FUNCTION "DIALOGO CON AP&T" : VOID
TITLE =Comunicazione AP&T
AUTHOR : D_T
FAMILY : DESTACK
NAME : COMUN
VERSION : 0.1


VAR_TEMP
  Klaschka_Alto : BOOL ;	//Klaschka Alto x Sicurezza movimentazione SMC
  BraccioAPT_FI : BOOL ;	//Braccio AP&T Fuori Ingombro da Pressa
END_VAR
BEGIN
NETWORK
TITLE =Per AP&T: Accensione motori
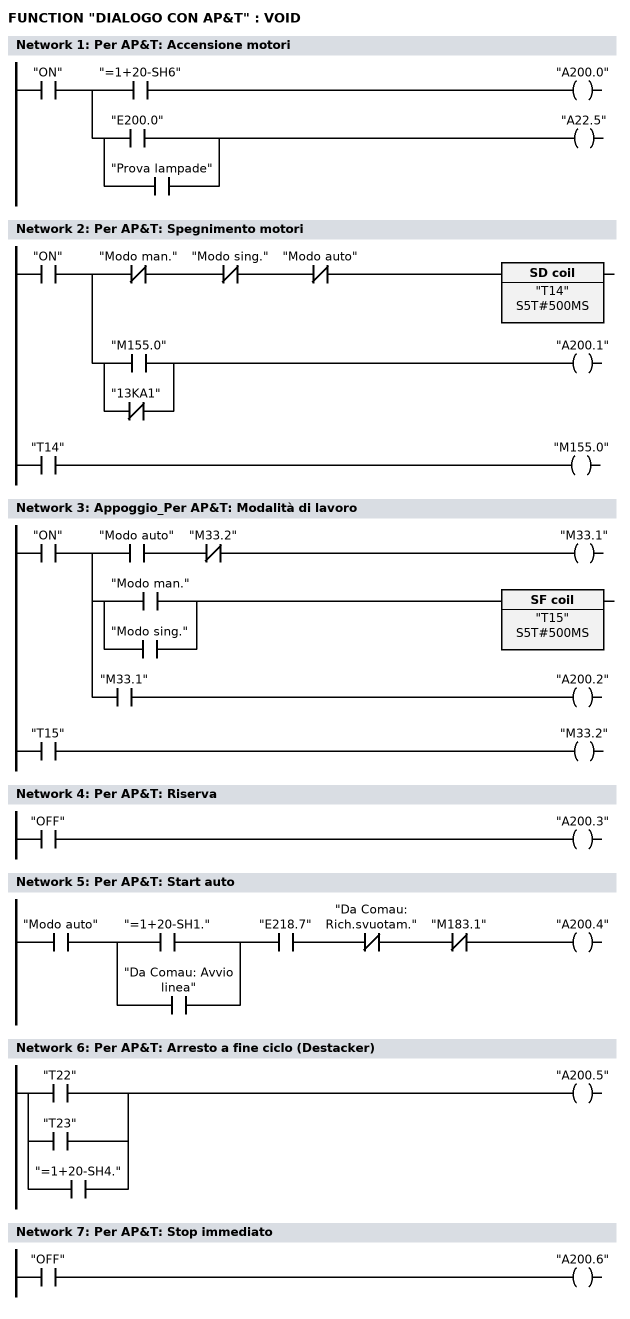
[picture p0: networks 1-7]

      U     "ON";
      =     L      1.0;
      U     L      1.0;
      U     "=1+20-SH6";
      =     "A200.0";
      U     L      1.0;
      U(    ;
      O     "E200.0";
      O     "Prova lampade";
      )     ;
      =     "A22.5";
NETWORK
TITLE =Per AP&T: Spegnimento motori

      U     "ON";
      =     L      1.0;
      U     L      1.0;
      UN    "Modo man.";
      UN    "Modo sing.";
      UN    "Modo auto";
      L     S5T#500MS;
      SE    "T14";
      NOP   0;
      NOP   0;
      NOP   0;
      U     "T14";
      =     "M155.0";
      U     L      1.0;
      U(    ;
      O     "M155.0";
      ON    "13KA1";
      )     ;
      =     "A200.1";
NETWORK
TITLE =Appoggio_Per AP&T: Modalità di lavoro

      U     "ON";
      =     L      1.0;
      U     L      1.0;
      U     "Modo auto";
      UN    "M33.2";
      =     "M33.1";
      U     L      1.0;
      U(    ;
      O     "Modo man.";
      O     "Modo sing.";
      )     ;
      L     S5T#500MS;
      SA    "T15";
      NOP   0;
      NOP   0;
      NOP   0;
      U     "T15";
      =     "M33.2";
      U     L      1.0;
      U     "M33.1";
      =     "A200.2";
NETWORK
TITLE =Per AP&T: Riserva

      U     "OFF";
      =     "A200.3";
NETWORK
TITLE =Per AP&T: Start auto

      U     "Modo auto";
      U(    ;
      O     "=1+20-SH1.";
      O     "Da Comau: Avvio linea";
      )     ;
      U     "E218.7";
      UN    "Da Comau: Rich.svuotam.";
      UN    "M183.1";
      =     "A200.4";
NETWORK
TITLE =Per AP&T: Arresto a fine ciclo (Destacker)

      O     "T22";
      O     "T23";
      O     "=1+20-SH4.";
      =     "A200.5";
NETWORK
TITLE =Per AP&T: Stop immediato

      U     "OFF";
      =     "A200.6";
NETWORK
TITLE =Per AP&T: Vai in posizione di cambio tooling

      U     "ON";
      =     L      1.0;
      U     L      1.0;
      U(    ;
      U     "AP&T in Manuale";
      U     "M130.5";
      O     ;
      U     "AP&T in Automatico";
      U     "Cambio produz. in corso";
      U     "Cambio prod.: Passo 7";
      )     ;
      =     L      1.1;
      U(    ;
      U     L      1.1;
      U     "Gruppi a riposo";
      U     "Magneti Indietro";
      UN    "Retrofitt. Ripari x AP&T";
      UN    "E200.1";
      L     S5T#2S;
      SE    "T59";
      NOP   0;
      NOP   0;
      NOP   0;
      U     "T59";
      )     ;
      FP    "M269.0";
      S     "A200.7";
      U     L      1.1;
      BLD   102;
      =     "Contr.gruppi a riposo";
      U     L      1.0;
      U     "A200.7";
      L     S5T#4S;
      SE    "T45";
      NOP   0;
      NOP   0;
      NOP   0;
      U     "T45";
      R     "A200.7";
NETWORK
TITLE =Per AP&T: Reset allarmi
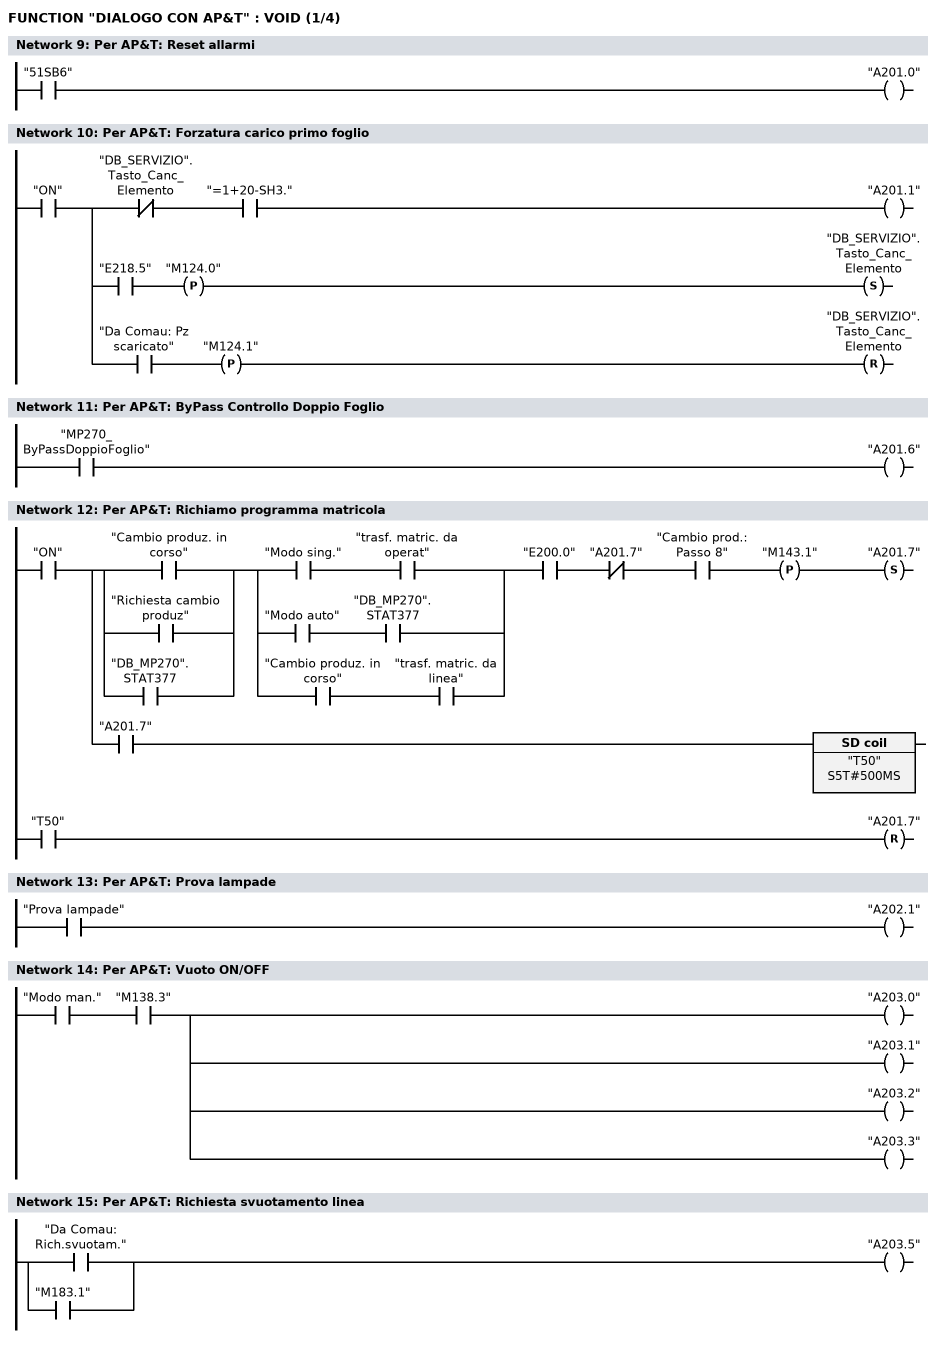
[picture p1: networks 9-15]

      U     "51SB6";
      =     "A201.0";
NETWORK
TITLE =Per AP&T: Forzatura carico primo foglio

      U     "ON";
      =     L      1.0;
      U     L      1.0;
      UN    "DB_SERVIZIO".Tasto_Canc_Elemento;
      U     "=1+20-SH3.";
      =     "A201.1";
      U     L      1.0;
      U     "E218.5";
      FP    "M124.0";
      S     "DB_SERVIZIO".Tasto_Canc_Elemento;
      U     L      1.0;
      U     "Da Comau: Pz scaricato";
      FP    "M124.1";
      R     "DB_SERVIZIO".Tasto_Canc_Elemento;
NETWORK
TITLE =Per AP&T: ByPass Controllo Doppio Foglio

      U     "MP270_ByPassDoppioFoglio";
      =     "A201.6";
NETWORK
TITLE =Per AP&T: Richiamo programma matricola

      U     "ON";
      =     L      1.0;
      U     L      1.0;
      U(    ;
      O     "Cambio produz. in corso";
      O     "Richiesta cambio produz";
      O     "DB_MP270".STAT377;
      )     ;
      U(    ;
      U     "Modo sing.";
      U     "trasf. matric. da operat";
      O     ;
      U     "Modo auto";
      U     "DB_MP270".STAT377;
      O     ;
      U     "Cambio produz. in corso";
      U     "trasf. matric. da linea";
      )     ;
      U     "E200.0";
      UN    "A201.7";
      U     "Cambio prod.: Passo 8";
      FP    "M143.1";
      S     "A201.7";
      U     L      1.0;
      U     "A201.7";
      L     S5T#500MS;
      SE    "T50";
      NOP   0;
      NOP   0;
      NOP   0;
      U     "T50";
      R     "A201.7";
NETWORK
TITLE =Per AP&T: Prova lampade

      U     "Prova lampade";
      =     "A202.1";
NETWORK
TITLE =Per AP&T: Vuoto ON/OFF

      U     "Modo man.";
      U     "M138.3";
      =     "A203.0";
      =     "A203.1";
      =     "A203.2";
      =     "A203.3";
NETWORK
TITLE =Per AP&T: Richiesta svuotamento linea

      O     "Da Comau: Rich.svuotam.";
      O     "M183.1";
      =     "A203.5";
NETWORK
TITLE =Per AP&T: Richiesta apertura
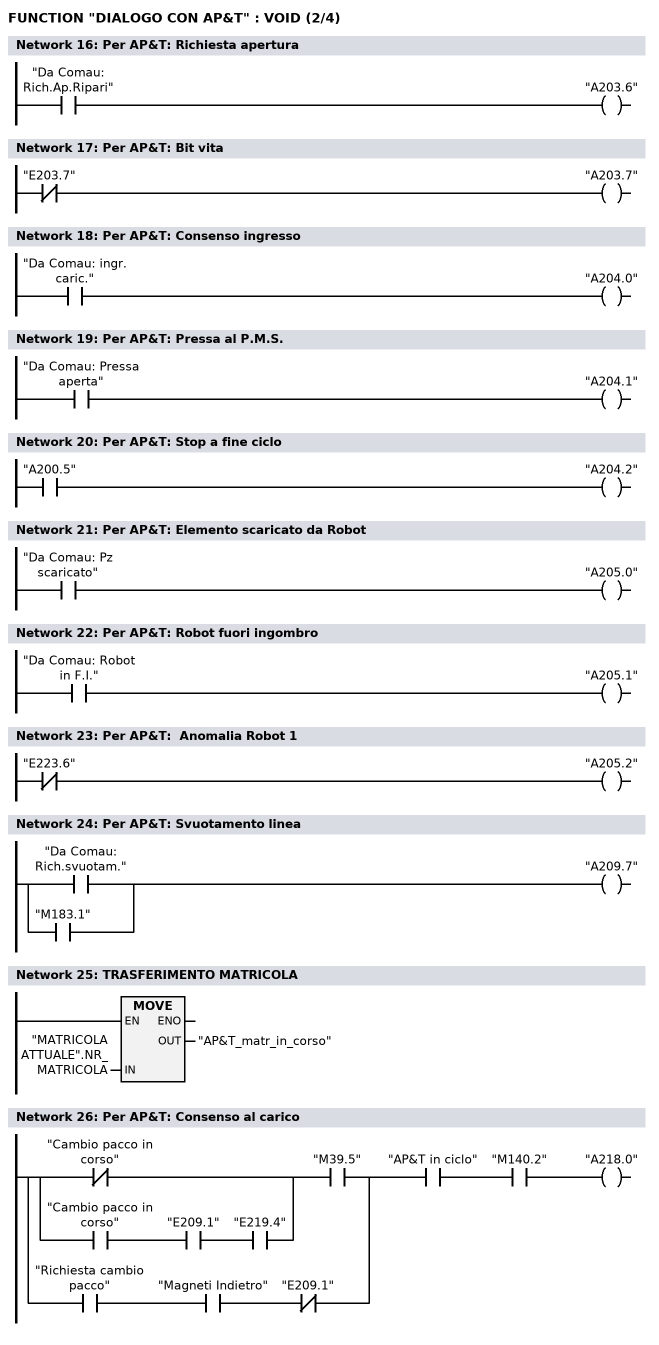
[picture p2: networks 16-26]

      U     "Da Comau: Rich.Ap.Ripari";
      =     "A203.6";
NETWORK
TITLE =Per AP&T: Bit vita

      UN    "E203.7";
      =     "A203.7";
NETWORK
TITLE =Per AP&T: Consenso ingresso

      U     "Da Comau: ingr. caric.";
      =     "A204.0";
NETWORK
TITLE =Per AP&T: Pressa al P.M.S.

      U     "Da Comau: Pressa aperta";
      =     "A204.1";
NETWORK
TITLE =Per AP&T: Stop a fine ciclo

      U     "A200.5";
      =     "A204.2";
NETWORK
TITLE =Per AP&T: Elemento scaricato da Robot

      U     "Da Comau: Pz scaricato";
      =     "A205.0";
NETWORK
TITLE =Per AP&T: Robot fuori ingombro

      U     "Da Comau: Robot in F.I.";
      =     "A205.1";
NETWORK
TITLE =Per AP&T:  Anomalia Robot 1

      UN    "E223.6";
      =     "A205.2";
NETWORK
TITLE =Per AP&T: Svuotamento linea

      O     "Da Comau: Rich.svuotam.";
      O     "M183.1";
      =     "A209.7";
NETWORK
TITLE =TRASFERIMENTO MATRICOLA

      L     "MATRICOLA ATTUALE".NR_MATRICOLA;
      T     "AP&T_matr_in_corso";
      NOP   0;
NETWORK
TITLE =Per AP&T: Consenso al carico

      U(    ;
      U(    ;
      ON    "Cambio pacco in corso";
      O     ;
      U     "Cambio pacco in corso";
      U     "E209.1";
      U     "E219.4";
      )     ;
      U     "M39.5";
      O     ;
      U     "Richiesta cambio pacco";
      U     "Magneti Indietro";
      UN    "E209.1";
      )     ;
      U     "AP&T in ciclo";
      U     "M140.2";
      =     "A218.0";
NETWORK
TITLE =Per AP&T: Prelievo foglio sfogliatore
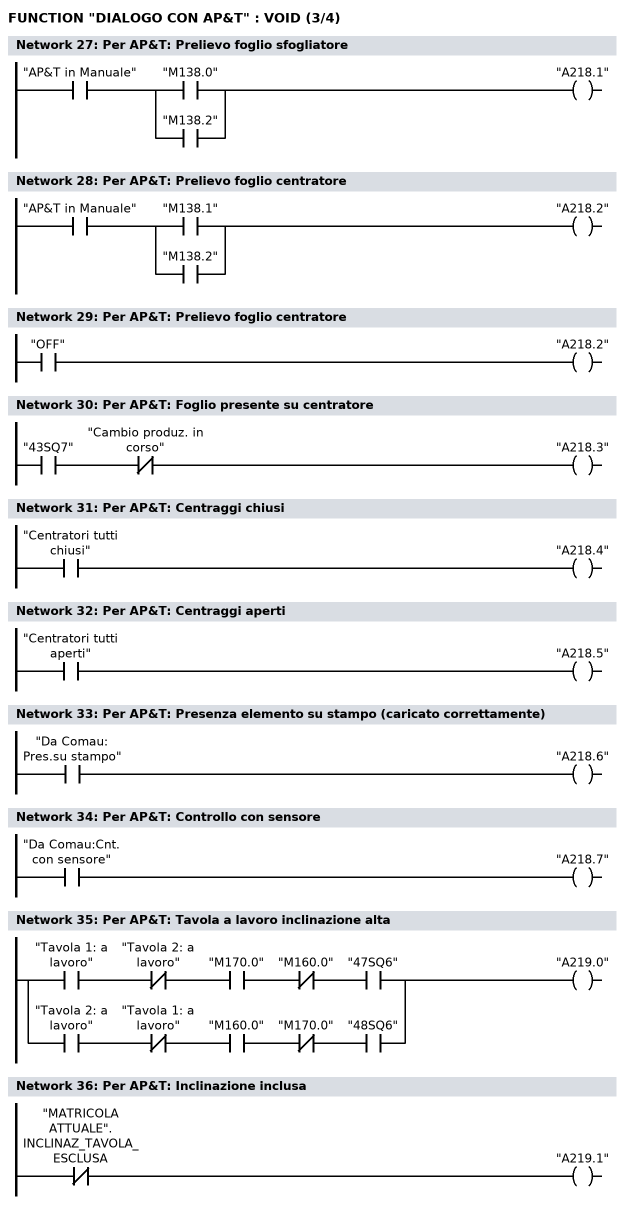
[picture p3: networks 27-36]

      U     "AP&T in Manuale";
      U(    ;
      O     "M138.0";
      O     "M138.2";
      )     ;
      =     "A218.1";
NETWORK
TITLE =Per AP&T: Prelievo foglio centratore

      U     "AP&T in Manuale";
      U(    ;
      O     "M138.1";
      O     "M138.2";
      )     ;
      =     "A218.2";
NETWORK
TITLE =Per AP&T: Prelievo foglio centratore

      U     "OFF";
      =     "A218.2";
NETWORK
TITLE =Per AP&T: Foglio presente su centratore

      U     "43SQ7";
      UN    "Cambio produz. in corso";
      =     "A218.3";
NETWORK
TITLE =Per AP&T: Centraggi chiusi

      U     "Centratori tutti chiusi";
      =     "A218.4";
NETWORK
TITLE =Per AP&T: Centraggi aperti

      U     "Centratori tutti aperti";
      =     "A218.5";
NETWORK
TITLE =Per AP&T: Presenza elemento su stampo (caricato correttamente)

      U     "Da Comau: Pres.su stampo";
      =     "A218.6";
NETWORK
TITLE =Per AP&T: Controllo con sensore

      U     "Da Comau:Cnt.con sensore";
      =     "A218.7";
NETWORK
TITLE =Per AP&T: Tavola a lavoro inclinazione alta

      U     "Tavola 1: a lavoro";
      UN    "Tavola 2: a lavoro";
      U     "M170.0";
      UN    "M160.0";
      U     "47SQ6";
      O     ;
      U     "Tavola 2: a lavoro";
      UN    "Tavola 1: a lavoro";
      U     "M160.0";
      UN    "M170.0";
      U     "48SQ6";
      =     "A219.0";
NETWORK
TITLE =Per AP&T: Inclinazione inclusa

      UN    "MATRICOLA ATTUALE".INCLINAZ_TAVOLA_ESCLUSA;
      =     "A219.1";
NETWORK
TITLE =Per AP&T: Tavole 1 o 2 sotto destacker
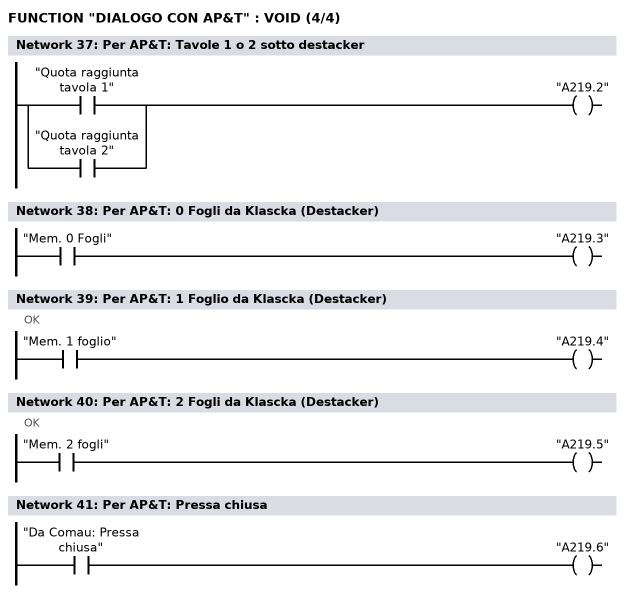
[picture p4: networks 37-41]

      O     "Quota raggiunta tavola 1";
      O     "Quota raggiunta tavola 2";
      =     "A219.2";
NETWORK
TITLE =Per AP&T: 0 Fogli da Klascka (Destacker)

      U     "Mem. 0 Fogli";
      =     "A219.3";
NETWORK
TITLE =Per AP&T: 1 Foglio da Klascka (Destacker)
//OK
      U     "Mem. 1 foglio";
      =     "A219.4";
NETWORK
TITLE =Per AP&T: 2 Fogli da Klascka (Destacker)
//OK
      U     "Mem. 2 fogli";
      =     "A219.5";
NETWORK
TITLE =Per AP&T: Pressa chiusa

      U     "Da Comau: Pressa chiusa";
      =     "A219.6";
NETWORK
TITLE =Per AP&T: Comando manuale home position

      U     "ON";
      =     L      1.0;
      U(    ;
      U     L      1.0;
      U(    ;
      O     "AP&T in Manuale";
      O     "AP&T in Automatico";
      )     ;
      U(    ;
      UN    "AP&T in Automatico";
      U     "M130.1";
      O     ;
      U(    ;
      O     "Cambio produz. in corso";
      O     "Richiesta cambio produz";
      )     ;
      U(    ;
      O     "Cambio prod.: Passo 1";
      O     "Cambio prod.: Passo 9";
      )     ;
      O     ;
      UN    "Cambio produz. in corso";
      UN    "Richiesta cambio produz";
      U     "Da Comau: Rich.Ap.Ripari";
      UN    "E219.7";
      )     ;
      UN    "E218.7";
      UN    "E200.1";
      L     S5T#2S;
      SE    "T58";
      NOP   0;
      NOP   0;
      NOP   0;
      U     "T58";
      )     ;
      FP    "M269.4";
      S     "A219.7";
      U     L      1.0;
      U     "A219.7";
      L     S5T#4S;
      SE    "T51";
      NOP   0;
      NOP   0;
      NOP   0;
      U     "T51";
      R     "A219.7";
NETWORK
TITLE =Per AP&T: Vai in posizione di Prelievo
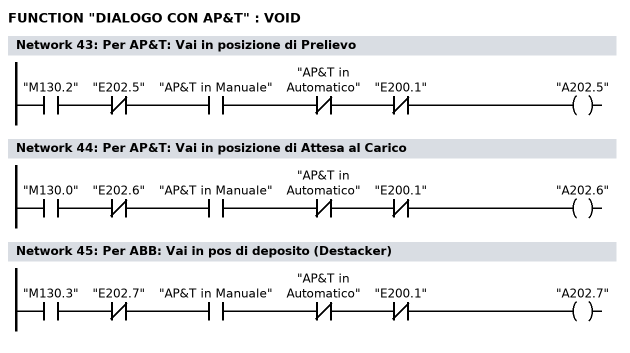
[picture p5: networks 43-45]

      U     "M130.2";
      UN    "E202.5";
      U     "AP&T in Manuale";
      UN    "AP&T in Automatico";
      UN    "E200.1";
      =     "A202.5";
NETWORK
TITLE =Per AP&T: Vai in posizione di Attesa al Carico

      U     "M130.0";
      UN    "E202.6";
      U     "AP&T in Manuale";
      UN    "AP&T in Automatico";
      UN    "E200.1";
      =     "A202.6";
NETWORK
TITLE =Per ABB: Vai in pos di deposito (Destacker)

      U     "M130.3";
      UN    "E202.7";
      U     "AP&T in Manuale";
      UN    "AP&T in Automatico";
      UN    "E200.1";
      =     "A202.7";
NETWORK
TITLE =Richiesta fine ciclo per apertura ripari o Klascka non OK
//OK
      U(    ;
      O     "61SA1";
      O     "61SA2";
      O     "61SA3";
      O     "61SA4";
      O     ;
      U(    ;
      UN    "Klascka 0 Fg.";
      UN    "Klascka 1 Fg.";
      UN    "Klascka 2 Fg.";
      L     S5T#10S;
      SE    "T4";
      NOP   0;
      NOP   0;
      NOP   0;
      U     "T4";
      )     ;
      U     "OFF";
      O     ;
      U     "AP&T in Automatico";
      U     "Richiesta cambio produz";
      U     "Cambio prod.: Passo 1";
      O     "Da Comau: Stop a Fine c.";
      O     "Da Comau: Stop linea";
      )     ;
      L     S5T#500MS;
      SV    "T22";
      NOP   0;
      NOP   0;
      NOP   0;
      NOP   0;
NETWORK
TITLE =Impulso richiesta apertura ripari
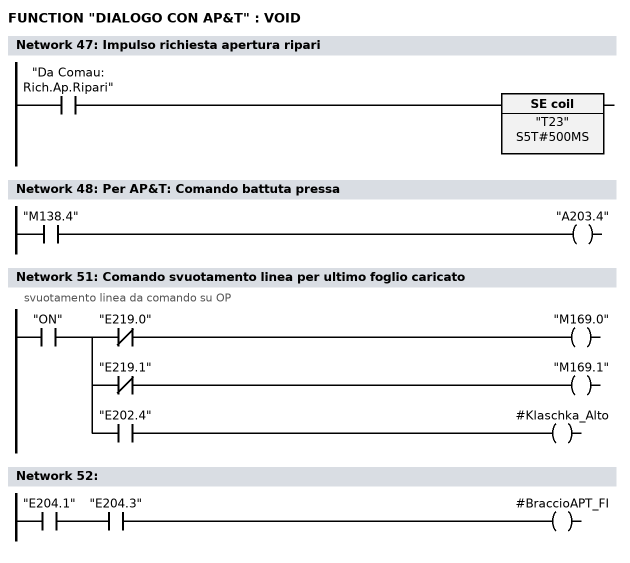
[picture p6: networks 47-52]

      U     "Da Comau: Rich.Ap.Ripari";
      L     S5T#500MS;
      SV    "T23";
      NOP   0;
      NOP   0;
      NOP   0;
      NOP   0;
NETWORK
TITLE =Per AP&T: Comando battuta pressa

      U     "M138.4";
      =     "A203.4";
NETWORK
TITLE =Klascka prox sicurezza salita

NETWORK
TITLE =Braccio AP&T Fuori Ingombro da Pressa

NETWORK
TITLE =Comando svuotamento linea per ultimo foglio caricato
//svuotamento linea da comando su OP
      U     "ON";
      =     L      1.0;
      U     L      1.0;
      UN    "E219.0";
      =     "M169.0";
      U     L      1.0;
      UN    "E219.1";
      =     "M169.1";
      U     L      1.0;
      U     "E202.4";
      =     #Klaschka_Alto;
NETWORK
TITLE =

      U     "E204.1";
      U     "E204.3";
      =     #BraccioAPT_FI;
NETWORK
TITLE =Timer

      UN    "VER";
      =     L      1.0;
      U(    ;
      U     L      1.0;
      U     "Modo auto";
      U     "M183.0";
      U     "AP&T in ciclo";
      U     "E209.1";
      U(    ;
      U     "Foglio_0";
      U     "OFF";
      O     "Mem. 0 Fogli";
      O     ;
      UN    "VER";
      UN    "Mem. 0 Fogli";
      U     "Da Comau: Rich.svuotam.";
      O     ;
      UN    "VER";
      U     "KEYENCE";
      )     ;
      L     S5T#5S;
      SE    "T100";
      NOP   0;
      NOP   0;
      NOP   0;
      U     "T100";
      )     ;
      FP    "M183.7";
      S     "M183.1";
      U     L      1.0;
      U     "M183.1";
      U     "E218.5";
      FP    "M183.2";
      SPBNB _001;
      L     1;
      L     "MW148";
      +I    ;
      T     "MW148";
_001: NOP   0;
      U     L      1.0;
      U(    ;
      O(    ;
      L     "MW148";
      L     1;
      >I    ;
      )     ;
      O(    ;
      L     "MW148";
      L     1;
      ==I   ;
      )     ;
      )     ;
      L     S5T#2S;
      SE    "T70";
      NOP   0;
      NOP   0;
      NOP   0;
      U     "T70";
      =     L      1.1;
      U     L      1.1;
      BLD   102;
      R     "M183.0";
      U     L      1.1;
      BLD   102;
      R     "M183.1";
      U     L      1.1;
      SPBNB _002;
      L     0;
      T     "MW148";
_002: NOP   0;
      U     L      1.0;
      UN    "M183.0";
      =     L      1.1;
      U     L      1.1;
      BLD   102;
      R     "M183.1";
      U     L      1.1;
      SPBNB _003;
      L     0;
      T     "MW148";
_003: NOP   0;
END_FUNCTION

